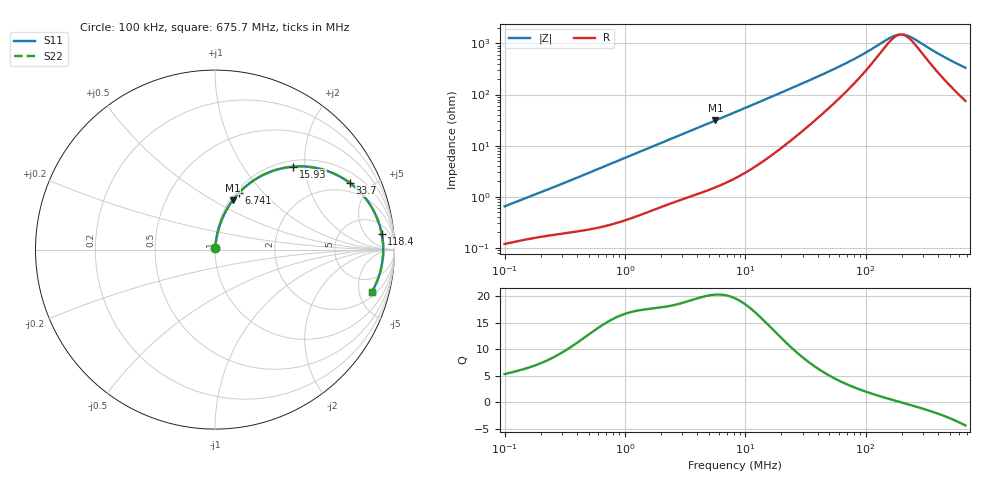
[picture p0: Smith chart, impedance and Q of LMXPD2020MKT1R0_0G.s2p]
! LMXPD2020MKT1R0_0G  S-PARAMETER MODEL  ( General Type )
! Model Generated by TAIYO YUDEN Corporation (https://www.yuden.co.jp/en/)
! Version 1.0
! TAIYO YUDEN Control No. 191023NI43SB-FBB
! Copyright(c) 2019 TAIYO YUDEN CO.,LTD. All Rights Reserved.
! Product Description (link to TY-COMPAS)
! https://ds.yuden.co.jp/TYCOMPAS/or/detail?pn=LMXPD2020MKT1R0N0G&u=M
! Products Name : Inductors
! Characteristics :
!  Inductance : 1.0 uH , SRF(min) : -Hz , DC Resistance(max) : 0.0876 Ohm
!  Rated Current : Saturation :2200 mA , Temp Rise : 1650 mA (40 degC)
!  Case Size : 2.0 x 2.0 / 0.079 x 0.079 [mm/inch] , Thickness : 1.2 / 0.047 [mm/inch]
!  (Conditions: Temperature = 25 degC , DC Bias Current/Voltage = 0A / 0V)
! External Node Assignments :
!  1  o---GGG---o  2
! GND o---------o GND
! Frequency Range : 0.1MHz  -  675.68652MHz  [ 402 STEP ]
# MHz S RI R 50
! Freq[MHz].  S11 Real  S11 Imag  S21 Real  S21 Imag  S12 Real  S12 Imag  S22 Real  S22 Imag
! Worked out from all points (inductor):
!   401 points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, 100 kHz to 675.7 MHz, reference 50 ohm
!   read as one part in series: L = 996 nH near 104.5 kHz
!   highest Q = 20.3 at 5.651 MHz (marker M1), where L = 874 nH
!   self-resonance near 197.4 MHz
!   S11 on the Smith chart (normalised r, x): 100 kHz: 1.00, +0.01; 6.741 MHz: 1.04, +0.74; 15.93 MHz: 1.12, +1.74; 33.7 MHz: 1.49, +3.72; 118.4 MHz: 10, +14; 675.7 MHz: 2.50, -6.53
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0.1  0.00123 0.00636  0.9988 -0.00636  0.9988 -0.00636  0.00123 0.00636
0.438008  0.00281 0.0256  0.9972 -0.0256  0.9972 -0.0256  0.00281 0.0256
0.990225  0.00661 0.0565  0.9934 -0.0565  0.9934 -0.0565  0.00661 0.0565
1.918513  0.0175 0.1059  0.9825 -0.1059  0.9825 -0.1059  0.0175 0.1059
3.556697  0.0465 0.1862  0.9535 -0.1862  0.9535 -0.1862  0.0465 0.1862
5.650781  0.0992 0.2754  0.9008 -0.2754  0.9008 -0.2754  0.0992 0.2754
6.740675  0.1321 0.3148  0.8679 -0.3148  0.8679 -0.3148  0.1321 0.3148
8.403244  0.1869 0.3651  0.8131 -0.3651  0.8131 -0.3651  0.1869 0.3651
11.9574  0.3099 0.4341  0.6901 -0.4341  0.6901 -0.4341  0.3099 0.4341
15.92588  0.4365 0.4624  0.5635 -0.4624  0.5635 -0.4624  0.4365 0.4624
22.66174  0.5996 0.4464  0.4004 -0.4464  0.4004 -0.4464  0.5996 0.4464
33.70015  0.7514 0.3714  0.2486 -0.3714  0.2486 -0.3714  0.7514 0.3714
36.00435  0.7714 0.3555  0.2286 -0.3555  0.2286 -0.3555  0.7714 0.3555
61.11385  0.8798 0.2238  0.1202 -0.2238  0.1202 -0.2238  0.8798 0.2238
86.96199  0.9139 0.1457  0.0861 -0.1457  0.0861 -0.1457  0.9139 0.1457
118.4051  0.9293 0.0864  0.0707 -0.0864  0.0707 -0.0864  0.9293 0.0864
157.702  0.9359 0.0369  0.0641 -0.0369  0.0641 -0.0369  0.9359 0.0369
188.1188  0.9374 0.00786  0.0626 -0.00786  0.0626 -0.00786  0.9374 0.00786
205.4611  0.9374 -0.00656  0.0626 0.00656  0.0626 0.00656  0.9374 -0.00656
224.4022  0.937 -0.021  0.063 0.021  0.063 0.021  0.937 -0.021
444.4597  0.9147 -0.1442  0.0853 0.1442  0.0853 0.1442  0.9147 -0.1442
675.6865  0.8724 -0.2382  0.1276 0.2382  0.1276 0.2382  0.8724 -0.2382
